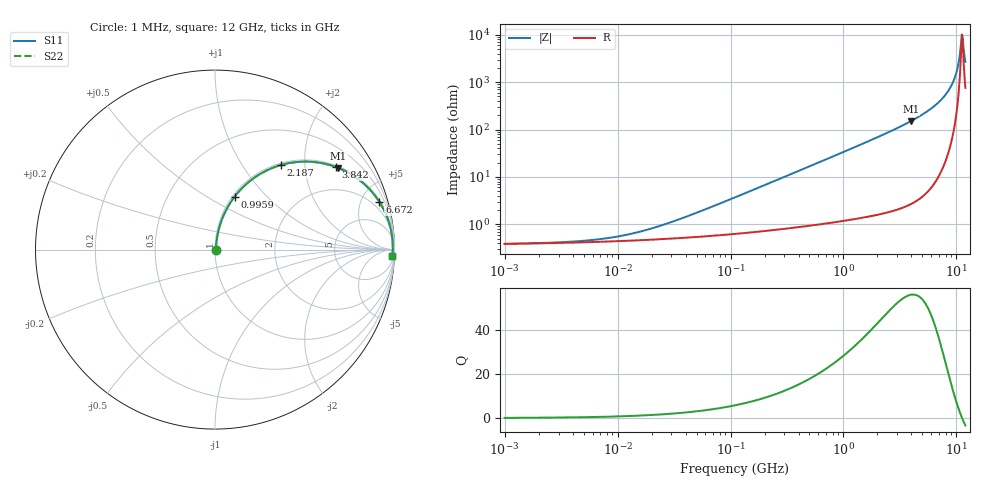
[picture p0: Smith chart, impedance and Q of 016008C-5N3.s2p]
# MHz S MA R 50
!Freq  MagS11  AngS11  MagS21  AngS21  MagS12  AngS12  MagS22  AngS22
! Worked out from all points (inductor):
!   801 points, 1 MHz to 12 GHz, reference 50 ohm
!   read as one part in series: L = 5.3 nH near 48.73 MHz
!   highest Q = 56.3 at 3.933 GHz (marker M1), where L = 6.04 nH
!   self-resonance near 11.18 GHz
!   S11 on the Smith chart (normalised r, x): 1 MHz: 1.01, +0.00; 995.9 MHz: 1.02, +0.67; 2.187 GHz: 1.03, +1.51; 3.842 GHz: 1.05, +2.90; 6.672 GHz: 1.17, +6.87; 12 GHz: 16, -51
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1  0.003854 4.9  0.9962 -0.0  0.9962 -0.0  0.003854 4.9
4.822396  0.004441 21.0  0.9959 -0.1  0.9959 -0.1  0.004441 21.0
10.84157  0.005697 38.9  0.9956 -0.2  0.9956 -0.2  0.005697 38.9
22.98406  0.009003 57.3  0.9952 -0.4  0.9952 -0.4  0.009003 57.3
110.8382  0.03719 78.2  0.9931 -2.1  0.9931 -2.1  0.03719 78.2
528.267  0.1723 77.0  0.9758 -9.9  0.9758 -9.9  0.1723 77.0
995.8598  0.3139 69.7  0.9385 -18.3  0.9385 -18.3  0.3139 69.7
1484.443  0.4447 62.0  0.8835 -26.4  0.8835 -26.4  0.4447 62.0
2186.904  0.5974 52.1  0.7889 -36.7  0.7889 -36.7  0.5974 52.1
2517.778  0.6553 47.9  0.7421 -40.9  0.7421 -40.9  0.6553 47.9
3842.205  0.8164 34.3  0.5631 -54.7  0.5631 -54.7  0.8164 34.3
3933.494  0.8242 33.5  0.5518 -55.5  0.5518 -55.5  0.8242 33.5
5275.37  0.9078 23.7  0.4024 -65.2  0.4024 -65.2  0.9078 23.7
6671.637  0.9538 16.1  0.2775 -72.5  0.2775 -72.5  0.9538 16.1
8050.374  0.9771 10.2  0.1769 -77.5  0.1769 -77.5  0.9771 10.2
9268.379  0.987 5.8  0.1018 -79.8  0.1018 -79.8  0.987 5.8
10062.28  0.9898 3.3  0.05836 -78.3  0.05836 -78.3  0.9898 3.3
10423.02  0.9904 2.2  0.04002 -75.0  0.04002 -75.0  0.9904 2.2
10796.69  0.9906 1.2  0.02233 -64.5  0.02233 -64.5  0.9906 1.2
11053.21  0.9905 0.5  0.01233 -39.4  0.01233 -39.4  0.9905 0.5
11449.47  0.99 -0.6  0.01463 46.7  0.01463 46.7  0.99 -0.6
12000  0.9888 -2.0  0.03713 71.4  0.03713 71.4  0.9888 -2.0
